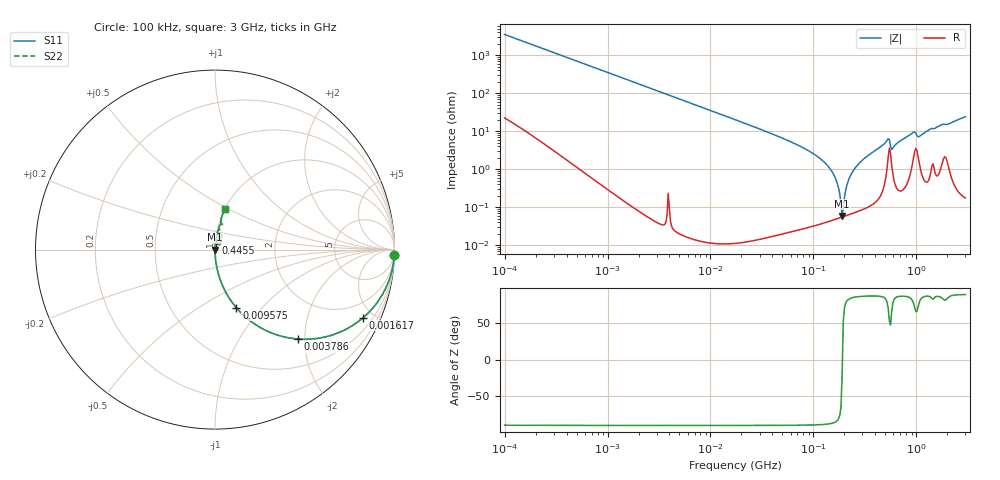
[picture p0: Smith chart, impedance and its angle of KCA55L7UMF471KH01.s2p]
!Murata Part Number: KCA55L7UMF471KH01
!These Parameters are Measured in Series Mode Connection
!Data Generated on Jan 08, 2026
!  o--ll--o
!Port1  Port2
!  o------o
!Operation Temp=25[degC], DC Bias Voltage=0[V]
!Freq. Start=100[kHz] Stop=3[GHz] 401[Steps]
# Hz S RI R 50
!Freq.(Hz) S11(Real) S11(Imag) S21(Real) S21(Imag) S12(Real) S12(Imag) S22(Real) S22(Imag)
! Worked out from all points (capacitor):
!   401 points, 100 kHz to 3 GHz, reference 50 ohm
!   read as one part in series: C = 452 pF near 105.3 kHz
!   lowest |Z| = 58.4 mohm at 190.3 MHz (marker M1)
!   series resonance near 191.4 MHz, so ESL is about 1.5 nH
!   S11 on the Smith chart (normalised r, x): 100 kHz: 1, -70; 1.617 MHz: 1.00, -4.36; 3.786 MHz: 1.00, -1.86; 9.575 MHz: 1.00, -0.73; 445.5 MHz: 1.00, +0.08; 3 GHz: 1.00, +0.48
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100000  0.999 -0.0284  0.000989 0.0284  0.000989 0.0284  0.999 -0.0284
562235  0.975 -0.1555  0.025 0.1555  0.025 0.1555  0.975 -0.1555
1617420  0.8258 -0.379  0.1742 0.379  0.1742 0.379  0.8258 -0.379
3161081  0.5539 -0.4969  0.4461 0.4969  0.4461 0.4969  0.5539 -0.4969
3786040  0.4635 -0.4983  0.5365 0.4983  0.5365 0.4983  0.4635 -0.4983
9574722  0.1188 -0.3234  0.8812 0.3234  0.8812 0.3234  0.1188 -0.3234
1.77727e7  0.0373 -0.1892  0.9627 0.1892  0.9627 0.1892  0.0373 -0.1892
9.738194e7  0.00103 -0.0267  0.999 0.0267  0.999 0.0267  0.00103 -0.0267
1.509232e8  0.000522 -0.0088  0.9995 0.0088  0.9995 0.0088  0.000522 -0.0088
1.673121e8  0.000512 -0.00495  0.9995 0.00495  0.9995 0.00495  0.000512 -0.00495
1.854806e8  0.000537 -0.00115  0.9995 0.00115  0.9995 0.00115  0.000537 -0.00115
1.90323e8  0.000549 -0.000199  0.9995 0.000199  0.9995 0.000199  0.000549 -0.000199
2.003904e8  0.000579 0.0017  0.9994 -0.0017  0.9994 -0.0017  0.000579 0.0017
2.164987e8  0.00064 0.00456  0.9994 -0.00456  0.9994 -0.00456  0.00064 0.00456
2.462744e8  0.00079 0.00942  0.9992 -0.00942  0.9992 -0.00942  0.00079 0.00942
4.455063e8  0.00335 0.0379  0.9967 -0.0379  0.9967 -0.0379  0.00335 0.0379
5.200087e8  0.0136 0.0549  0.9864 -0.0549  0.9864 -0.0549  0.0136 0.0549
5.475153e8  0.0368 0.0447  0.9632 -0.0447  0.9632 -0.0447  0.0368 0.0447
5.915271e8  0.00876 0.0344  0.9912 -0.0344  0.9912 -0.0344  0.00876 0.0344
9.167529e8  0.021 0.086  0.979 -0.086  0.979 -0.086  0.021 0.086
1.070062e9  0.0187 0.069  0.9813 -0.069  0.9813 -0.069  0.0187 0.069
3e9  0.0563 0.2269  0.9437 -0.2269  0.9437 -0.2269  0.0563 0.2269
